(* Logix 5000 AddOnInstructionDefinition export CIP_Axis_Disable; software revision 34.01 *)

TYPE CIP_Axis :   // CIP Sync Axis Object
STRUCT
   Control : CIP_Control;   // Control bits to send to the drive
   Status : CIP_Status;   // Status bits received from the drive
   Input : CIP_AxisInputData;   // Data from the drive
   Output : CIP_AxisOutputData;   // Data to the drive
   PositionFeedback : DINT;   // Actual Position Value
   PositionCommand : DINT;   // Drive's commanded position
   ResponseTimestamp : LINT;   // Drive's timestamp of response
   RequestedAction : INT;   // State_Machine_Requested_Action
END_STRUCT
END_TYPE

TYPE CIP_AxisInputData :
STRUCT
   Data : SINT[10];
END_STRUCT
END_TYPE

TYPE CIP_AxisOutputData :
STRUCT
   Data : SINT[14];
END_STRUCT
END_TYPE

TYPE CIP_Control :
STRUCT
   Switch_On : BOOL;
   Disable_Voltage : BOOL;
   Quick_Stop : BOOL;
   Enable_Operation : BOOL;
   Op_Mode_Specific_4 : BOOL;   // Home Start or Follow Position bit, depending on on whether bit 11 (Mode Home) or bit 12 (C
   Op_Mode_Specific_5 : BOOL;   // Unused
   Op_Mode_Specific_6 : BOOL;   // Unused
   Reset_Fault : BOOL;
   Pause_Halt : BOOL;
   Op_Mode_Specific_9 : BOOL;   // Unused
   Reserved_10 : BOOL;
   Manu_Specific_11 : BOOL;   // Mode Home bit
   Manu_Specific_12 : BOOL;   // Mode Cyclic Position bit
   Manu_Specific_13 : BOOL;   // Unused
   Manu_Specific_14 : BOOL;   // Unused
   Manu_Specific_15 : BOOL;   // Unused
END_STRUCT
END_TYPE

TYPE CIP_DynamicMap :
STRUCT
   Input : CIP_MapInputData;   // Map data from the drive
   Output : CIP_MapOutputData;   // Map data to the drive
END_STRUCT
END_TYPE

TYPE CIP_MapInputData :   // Map data received from the drive
STRUCT
   Data : SINT[40];
END_STRUCT
END_TYPE

TYPE CIP_MapOutputData :   // Map data going to drive
STRUCT
   Data : SINT[32];
END_STRUCT
END_TYPE

TYPE CIP_Status :   // All connections to the drive ethernet module are established and data is successfully transferring.
STRUCT
   Ready_To_Switch_On : BOOL;
   Switched_On : BOOL;
   Operation_Enabled : BOOL;
   Fault : BOOL;
   Voltage_Enabled : BOOL;
   Quick_Stop : BOOL;
   Switch_On_Disabled : BOOL;
   Warning : BOOL;
   STO_Active : BOOL;
   Remote : BOOL;
   Target_Reached : BOOL;
   Internal_Limit_Active : BOOL;
   Op_Mode_Specific_12 : BOOL;   // Home Attained bit
   Op_Mode_Specific_13 : BOOL;   // Homing/Cyclic Position Error bit
   Manu_Specific_14 : BOOL;   // Motion Mode bit (0 for Homing, 1 for Cyclic Position)
   Manu_Specific_15 : BOOL;   // Following Position bit (for Cyclic Position mode)
END_STRUCT
END_TYPE

ADD_ON_INSTRUCTION CIP_Axis_Disable   (* revision 2.1, ExecutePrescan, ExecuteEnableInFalse *)
// Disable CIP Sync Axis
VAR_OUTPUT
   DN : BOOL; {access Read Only, visible}   // Command Successful
   ER : BOOL; {access Read Only, visible}   // Error
END_VAR
VAR_IN_OUT
   Axis : CIP_Axis; {required}
END_VAR
VAR_OUTPUT
   Error_Code : SINT; {access Read Only, visible}
END_VAR
VAR_IN_OUT
   Error_Description : STRING; {required}
END_VAR
VAR
   CommandTimeout : TIMER;   // Timeout Timer
   Step : SINT; {access None}
   ErrorEnumeratedValues : STRING[2] := ([0] := 'No Error', [1] := 'Command Timeout'); {access None}
END_VAR

ROUTINE EnableInFalse   (* ladder *)
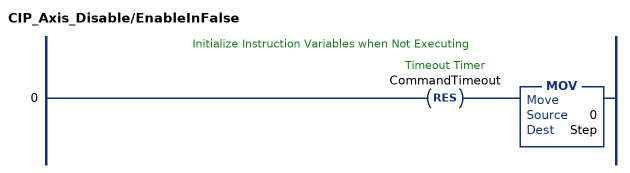
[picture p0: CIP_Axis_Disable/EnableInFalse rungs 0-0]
   // Initialize Instruction Variables when Not Executing
   0: RES(CommandTimeout)MOV(0,Step);
END_ROUTINE

ROUTINE Logic   (* ladder *)
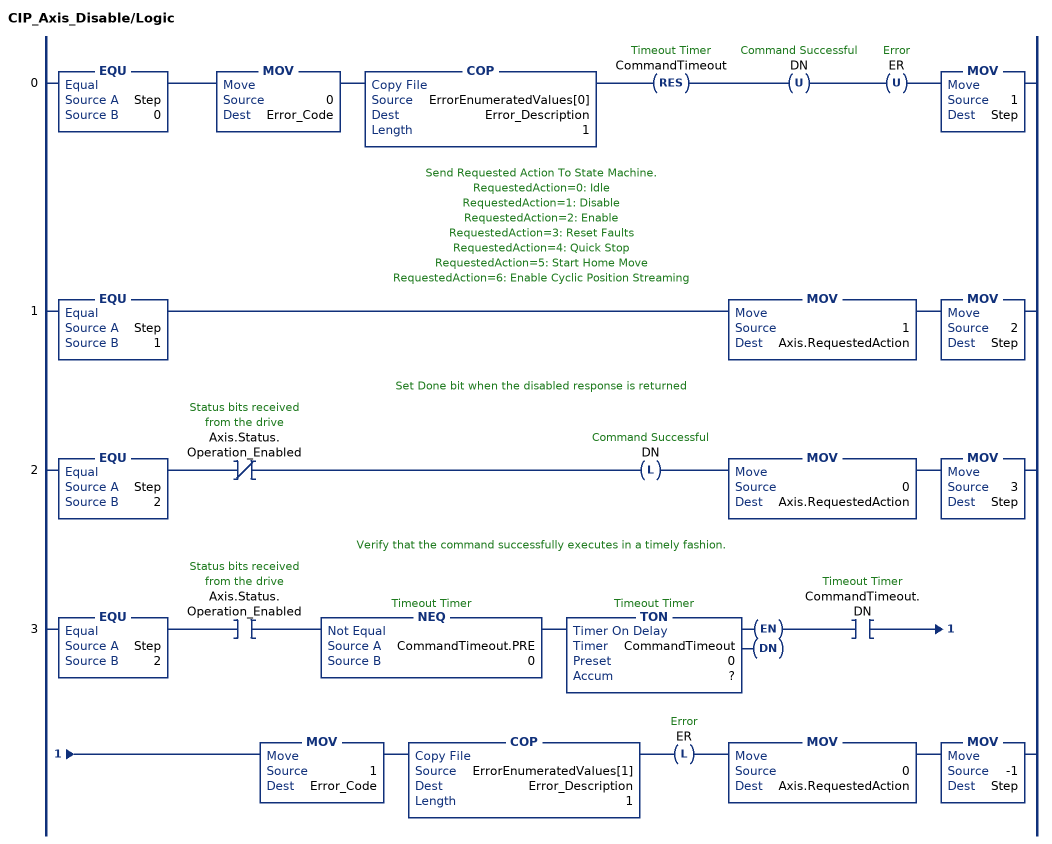
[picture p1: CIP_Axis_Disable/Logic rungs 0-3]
   0: EQU(Step,0)MOV(0,Error_Code)COP(ErrorEnumeratedValues[0],Error_Description,1)RES(CommandTimeout)OTU(DN)OTU(ER)MOV(1,Step);
   // Send Requested Action To State Machine.
   // RequestedAction=0: Idle
   // RequestedAction=1: Disable
   // RequestedAction=2: Enable
   // RequestedAction=3: Reset Faults
   // RequestedAction=4: Quick Stop
   // RequestedAction=5: Start Home Move
   // RequestedAction=6: Enable Cyclic Position Streaming
   1: EQU(Step,1)MOV(1,Axis.RequestedAction)MOV(2,Step);
   // Set Done bit when the disabled response is returned
   2: EQU(Step,2)XIO(Axis.Status.Operation_Enabled)OTL(DN)MOV(0,Axis.RequestedAction)MOV(3,Step);
   // Verify that the command successfully executes in a timely fashion.
   3: EQU(Step,2)XIC(Axis.Status.Operation_Enabled)NEQ(CommandTimeout.PRE,0)TON(CommandTimeout,?,?)XIC(CommandTimeout.DN)MOV(1,Error_Code)COP(ErrorEnumeratedValues[1],Error_Description,1)OTL(ER)MOV(0,Axis.RequestedAction)MOV(-1,Step);
END_ROUTINE

ROUTINE Prescan   (* ladder *)
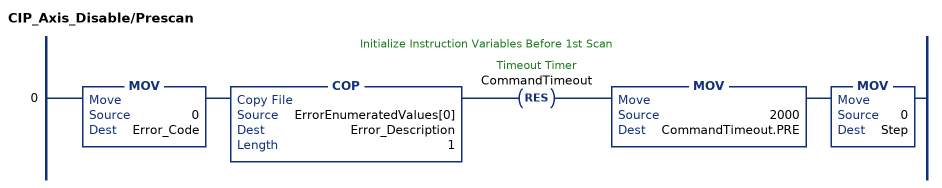
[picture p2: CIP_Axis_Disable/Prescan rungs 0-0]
   // Initialize Instruction Variables Before 1st Scan
   0: MOV(0,Error_Code)COP(ErrorEnumeratedValues[0],Error_Description,1)RES(CommandTimeout)MOV(2000,CommandTimeout.PRE)MOV(0,Step);
END_ROUTINE
END_ADD_ON_INSTRUCTION

ADD_ON_INSTRUCTION CIP_Axis_Disable_Streaming   (* revision 2.1, ExecutePrescan, ExecuteEnableInFalse *)
// CIP Sync Axis Disable Streaming
VAR_OUTPUT
   DN : BOOL; {access Read Only, visible}   // Command Successful
   ER : BOOL; {access Read Only, visible}   // Error
END_VAR
VAR_IN_OUT
   Axis : CIP_Axis; {required}
END_VAR
VAR_OUTPUT
   Error_Code : SINT; {access Read Only, visible}
END_VAR
VAR_IN_OUT
   Error_Description : STRING; {required}
END_VAR
VAR
   CommandTimeout : TIMER := (PRE := 2000); {access None}   // Timeout Timer
   Step : SINT; {access None}
   ErrorEnumeratedValues : STRING[2] := ([0] := 'No Error', [1] := 'Command Timeout'); {access None}
END_VAR

ROUTINE EnableInFalse   (* ladder *)
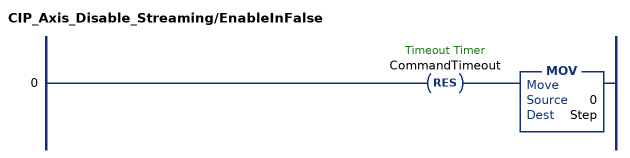
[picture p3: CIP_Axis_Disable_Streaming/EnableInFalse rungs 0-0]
   0: RES(CommandTimeout)MOV(0,Step);
END_ROUTINE

ROUTINE Logic   (* ladder *)
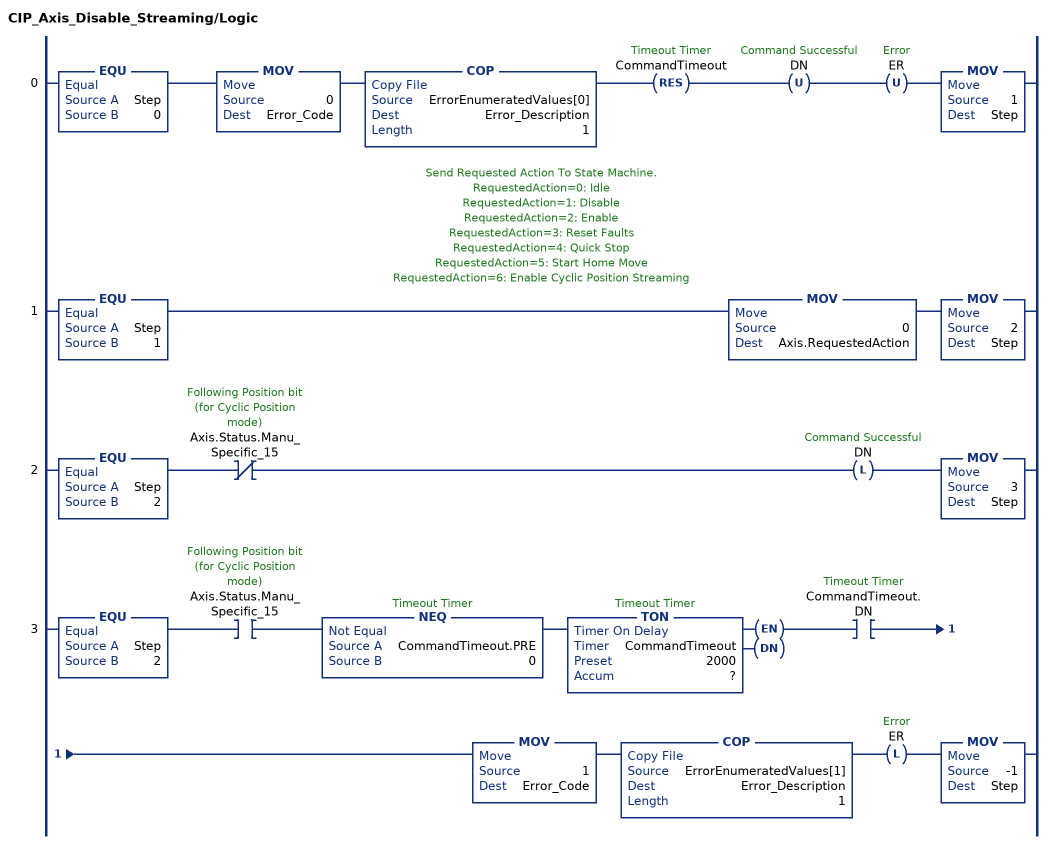
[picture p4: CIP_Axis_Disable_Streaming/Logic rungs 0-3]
   0: EQU(Step,0)MOV(0,Error_Code)COP(ErrorEnumeratedValues[0],Error_Description,1)RES(CommandTimeout)OTU(DN)OTU(ER)MOV(1,Step);
   // Send Requested Action To State Machine.
   // RequestedAction=0: Idle
   // RequestedAction=1: Disable
   // RequestedAction=2: Enable
   // RequestedAction=3: Reset Faults
   // RequestedAction=4: Quick Stop
   // RequestedAction=5: Start Home Move
   // RequestedAction=6: Enable Cyclic Position Streaming
   1: EQU(Step,1)MOV(0,Axis.RequestedAction)MOV(2,Step);
   2: EQU(Step,2)XIO(Axis.Status.Manu_Specific_15)OTL(DN)MOV(3,Step);
   3: EQU(Step,2)XIC(Axis.Status.Manu_Specific_15)NEQ(CommandTimeout.PRE,0)TON(CommandTimeout,?,?)XIC(CommandTimeout.DN)MOV(1,Error_Code)COP(ErrorEnumeratedValues[1],Error_Description,1)OTL(ER)MOV(-1,Step);
END_ROUTINE

ROUTINE Prescan   (* ladder *)
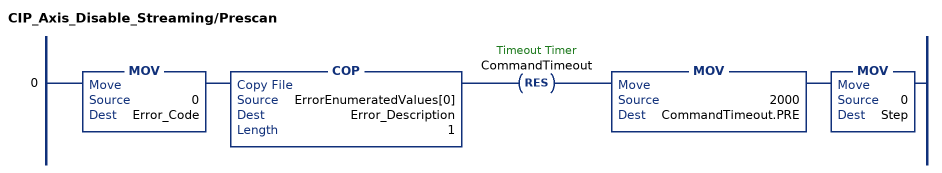
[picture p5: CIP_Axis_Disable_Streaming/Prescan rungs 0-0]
   0: MOV(0,Error_Code)COP(ErrorEnumeratedValues[0],Error_Description,1)RES(CommandTimeout)MOV(2000,CommandTimeout.PRE)MOV(0,Step);
END_ROUTINE
END_ADD_ON_INSTRUCTION

ADD_ON_INSTRUCTION CIP_Axis_Enable   (* revision 2.1, ExecutePrescan, ExecuteEnableInFalse *)
// Enables CIP Sync Axis
// Revision note:
// Bugfix: Added check of Axis.Status.Quick_Stop bit for confirming completion
VAR_OUTPUT
   DN : BOOL; {access Read Only, visible}   // Command Successful
   ER : BOOL; {access Read Only, visible}   // Error
END_VAR
VAR_IN_OUT
   Axis : CIP_Axis; {required}
END_VAR
VAR_OUTPUT
   Error_Code : SINT; {access Read Only, visible}
END_VAR
VAR_IN_OUT
   Error_Description : STRING; {required}
END_VAR
VAR
   CommandTimeout : TIMER := (PRE := 2000);   // Timeout Timer
   Step : SINT; {access None}
   ErrorEnumeratedValues : STRING[3] := ([0] := 'No Error', [1] := 'Command Timeout', [2] := 'Axis Faulted'); {access None}
END_VAR

ROUTINE EnableInFalse   (* ladder *)
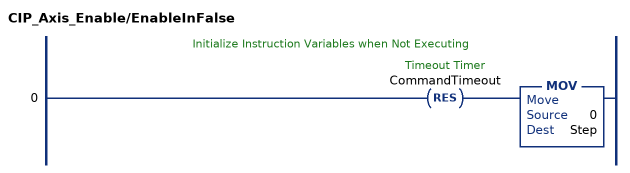
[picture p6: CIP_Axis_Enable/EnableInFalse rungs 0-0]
   // Initialize Instruction Variables when Not Executing
   0: RES(CommandTimeout)MOV(0,Step);
END_ROUTINE

ROUTINE Logic   (* ladder *)
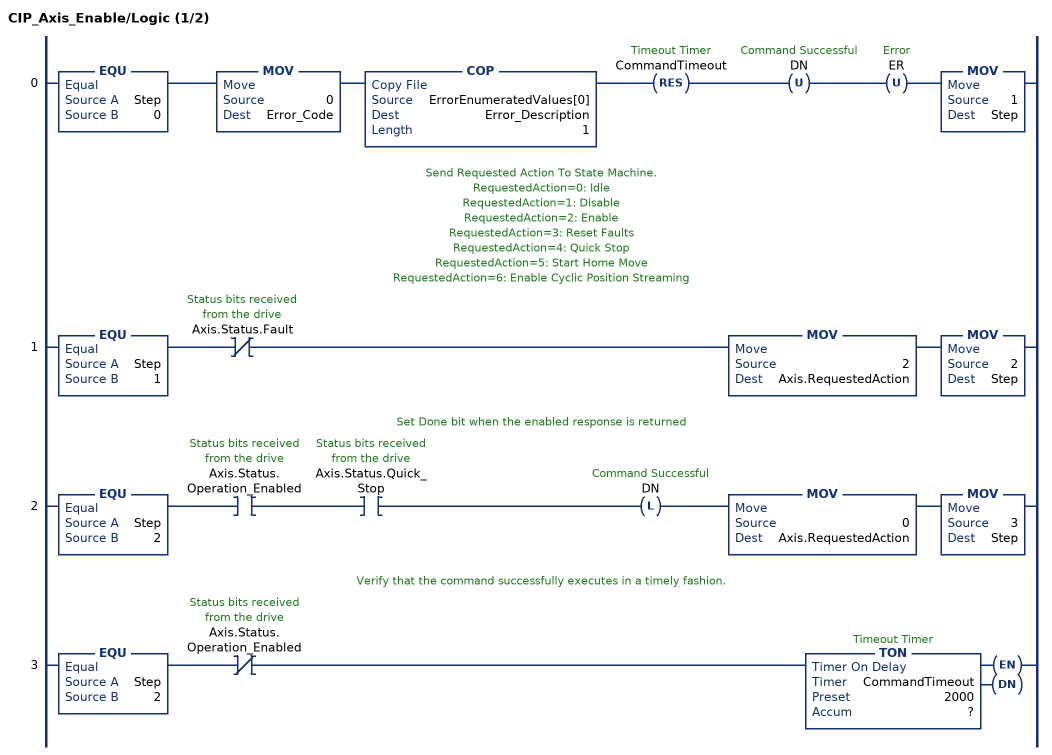
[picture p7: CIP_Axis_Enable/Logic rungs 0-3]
   0: EQU(Step,0)MOV(0,Error_Code)COP(ErrorEnumeratedValues[0],Error_Description,1)RES(CommandTimeout)OTU(DN)OTU(ER)MOV(1,Step);
   // Send Requested Action To State Machine.
   // RequestedAction=0: Idle
   // RequestedAction=1: Disable
   // RequestedAction=2: Enable
   // RequestedAction=3: Reset Faults
   // RequestedAction=4: Quick Stop
   // RequestedAction=5: Start Home Move
   // RequestedAction=6: Enable Cyclic Position Streaming
   1: EQU(Step,1)XIO(Axis.Status.Fault)MOV(2,Axis.RequestedAction)MOV(2,Step);
   // Set Done bit when the enabled response is returned
   2: EQU(Step,2)XIC(Axis.Status.Operation_Enabled)XIC(Axis.Status.Quick_Stop)OTL(DN)MOV(0,Axis.RequestedAction)MOV(3,Step);
   // Verify that the command successfully executes in a timely fashion.
   3: EQU(Step,2)XIO(Axis.Status.Operation_Enabled)TON(CommandTimeout,?,?);
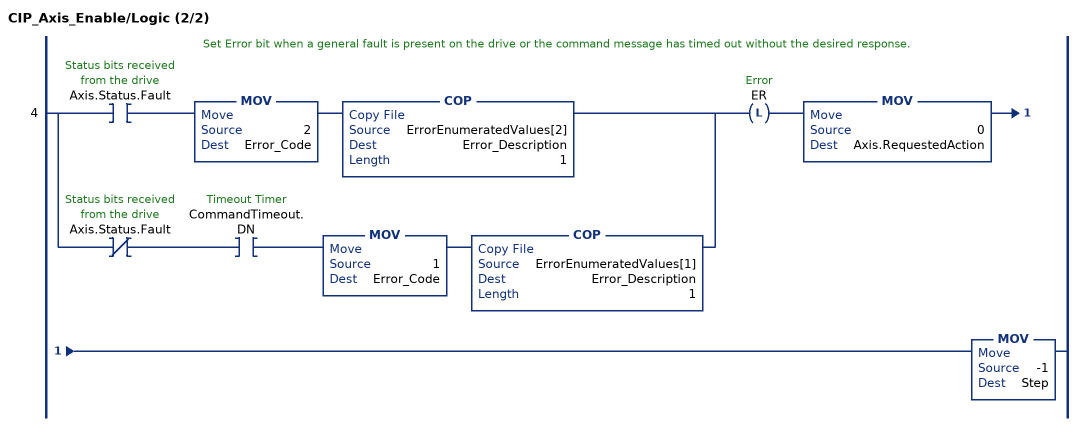
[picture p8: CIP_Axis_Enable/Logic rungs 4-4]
   // Set Error bit when a general fault is present on the drive or the command message has timed out without the desired response.
   4: [XIC(Axis.Status.Fault) MOV(2,Error_Code) COP(ErrorEnumeratedValues[2],Error_Description,1) ,XIO(Axis.Status.Fault) XIC(CommandTimeout.DN) MOV(1,Error_Code) COP(ErrorEnumeratedValues[1],Error_Description,1) ]OTL(ER)MOV(0,Axis.RequestedAction)MOV(-1,Step);
END_ROUTINE

ROUTINE Prescan   (* ladder *)
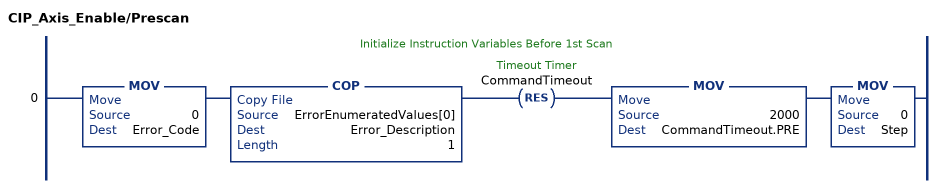
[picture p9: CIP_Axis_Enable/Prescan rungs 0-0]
   // Initialize Instruction Variables Before 1st Scan
   0: MOV(0,Error_Code)COP(ErrorEnumeratedValues[0],Error_Description,1)RES(CommandTimeout)MOV(2000,CommandTimeout.PRE)MOV(0,Step);
END_ROUTINE
END_ADD_ON_INSTRUCTION

ADD_ON_INSTRUCTION CIP_Axis_Enable_Streaming   (* revision 2.1, ExecutePrescan, ExecuteEnableInFalse *)
// CIP Sync Axis Enable Streaming
VAR_OUTPUT
   DN : BOOL; {access Read Only, visible}   // Command Successful
   ER : BOOL; {access Read Only, visible}   // Error
END_VAR
VAR_IN_OUT
   Axis : CIP_Axis; {required}
END_VAR
VAR_OUTPUT
   Error_Code : SINT; {visible}
END_VAR
VAR_IN_OUT
   Error_Description : STRING; {required}
END_VAR
VAR
   CommandTimeout : TIMER := (PRE := 2000); {access None}   // Timeout Timer
   Step : SINT; {access None}
   ErrorEnumeratedValues : STRING[5] := ([0] := 'No Error', [1] := 'Command Timeout', [2] := 'Axis Faulted', [3] := 'Home Not Attained', [4] := 'Axis Not Enabled'); {access None}
END_VAR

ROUTINE EnableInFalse   (* ladder *)
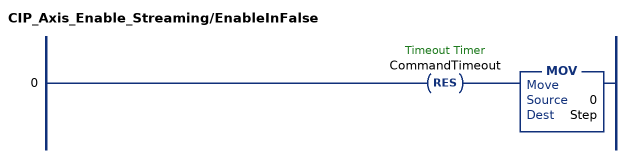
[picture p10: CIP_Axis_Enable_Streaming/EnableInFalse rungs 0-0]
   0: RES(CommandTimeout)MOV(0,Step);
END_ROUTINE

ROUTINE Logic   (* ladder *)
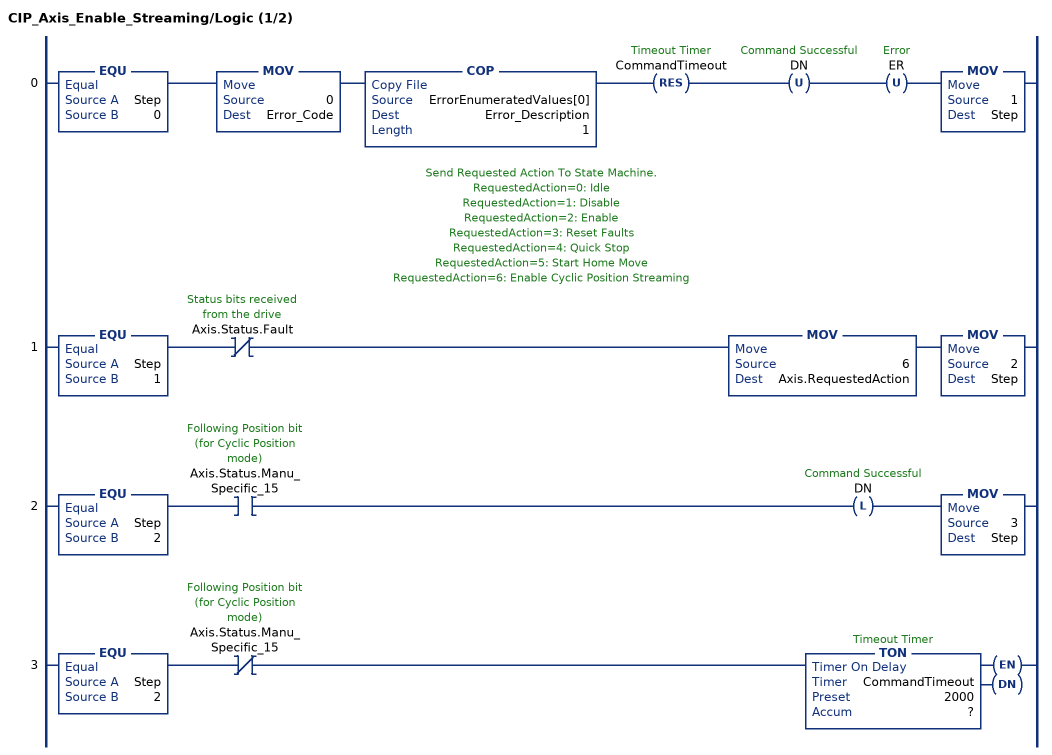
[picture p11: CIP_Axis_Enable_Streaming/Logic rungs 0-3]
   0: EQU(Step,0)MOV(0,Error_Code)COP(ErrorEnumeratedValues[0],Error_Description,1)RES(CommandTimeout)OTU(DN)OTU(ER)MOV(1,Step);
   // Send Requested Action To State Machine.
   // RequestedAction=0: Idle
   // RequestedAction=1: Disable
   // RequestedAction=2: Enable
   // RequestedAction=3: Reset Faults
   // RequestedAction=4: Quick Stop
   // RequestedAction=5: Start Home Move
   // RequestedAction=6: Enable Cyclic Position Streaming
   1: EQU(Step,1)XIO(Axis.Status.Fault)MOV(6,Axis.RequestedAction)MOV(2,Step);
   2: EQU(Step,2)XIC(Axis.Status.Manu_Specific_15)OTL(DN)MOV(3,Step);
   3: EQU(Step,2)XIO(Axis.Status.Manu_Specific_15)TON(CommandTimeout,?,?);
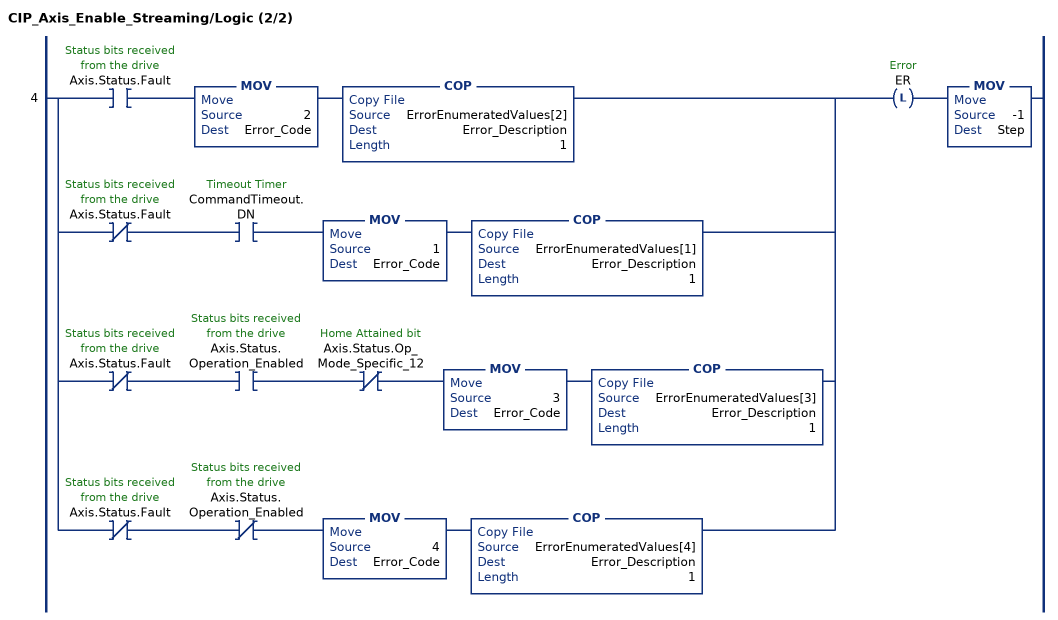
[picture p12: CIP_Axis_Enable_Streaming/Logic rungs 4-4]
   4: [XIC(Axis.Status.Fault) MOV(2,Error_Code) COP(ErrorEnumeratedValues[2],Error_Description,1) ,XIO(Axis.Status.Fault) XIC(CommandTimeout.DN) MOV(1,Error_Code) COP(ErrorEnumeratedValues[1],Error_Description,1) ,XIO(Axis.Status.Fault) XIC(Axis.Status.Operation_Enabled) XIO(Axis.Status.Op_Mode_Specific_12) MOV(3,Error_Code) COP(ErrorEnumeratedValues[3],Error_Description,1) ,XIO(Axis.Status.Fault) XIO(Axis.Status.Operation_Enabled) MOV(4,Error_Code) COP(ErrorEnumeratedValues[4],Error_Description,1) ]OTL(ER)MOV(-1,Step);
END_ROUTINE

ROUTINE Prescan   (* ladder *)
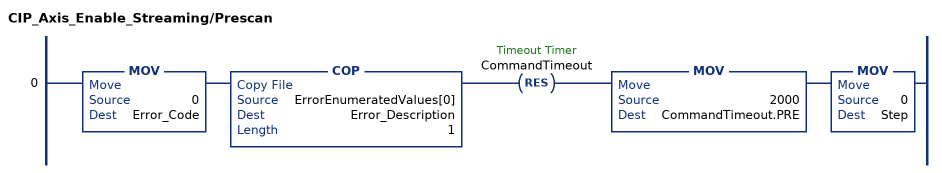
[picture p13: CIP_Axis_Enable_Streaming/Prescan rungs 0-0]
   0: MOV(0,Error_Code)COP(ErrorEnumeratedValues[0],Error_Description,1)RES(CommandTimeout)MOV(2000,CommandTimeout.PRE)MOV(0,Step);
END_ROUTINE
END_ADD_ON_INSTRUCTION

ADD_ON_INSTRUCTION CIP_Axis_Fault_Reset   (* revision 2.1, ExecutePrescan, ExecuteEnableInFalse *)
// CIP Sync Axis Fault Reset
VAR_OUTPUT
   DN : BOOL; {access Read Only, visible}   // Command Successful
   ER : BOOL; {access Read Only, visible}   // Error
END_VAR
VAR_IN_OUT
   Axis : CIP_Axis; {required}
END_VAR
VAR_OUTPUT
   Error_Code : SINT; {access Read Only, visible}
END_VAR
VAR_IN_OUT
   Error_Description : STRING; {required}
END_VAR
VAR
   Step : SINT;
   CommandTimeout : TIMER := (PRE := 2000); {access None}
   ErrorEnumeratedValues : STRING[2] := ([0] := 'No Error', [1] := 'Command Timeout'); {access None}
END_VAR

ROUTINE EnableInFalse   (* ladder *)
// EnableIn_False
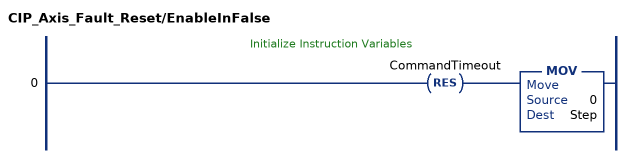
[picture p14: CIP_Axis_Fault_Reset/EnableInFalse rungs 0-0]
   // Initialize Instruction Variables
   0: RES(CommandTimeout)MOV(0,Step);
END_ROUTINE

ROUTINE Logic   (* ladder *)
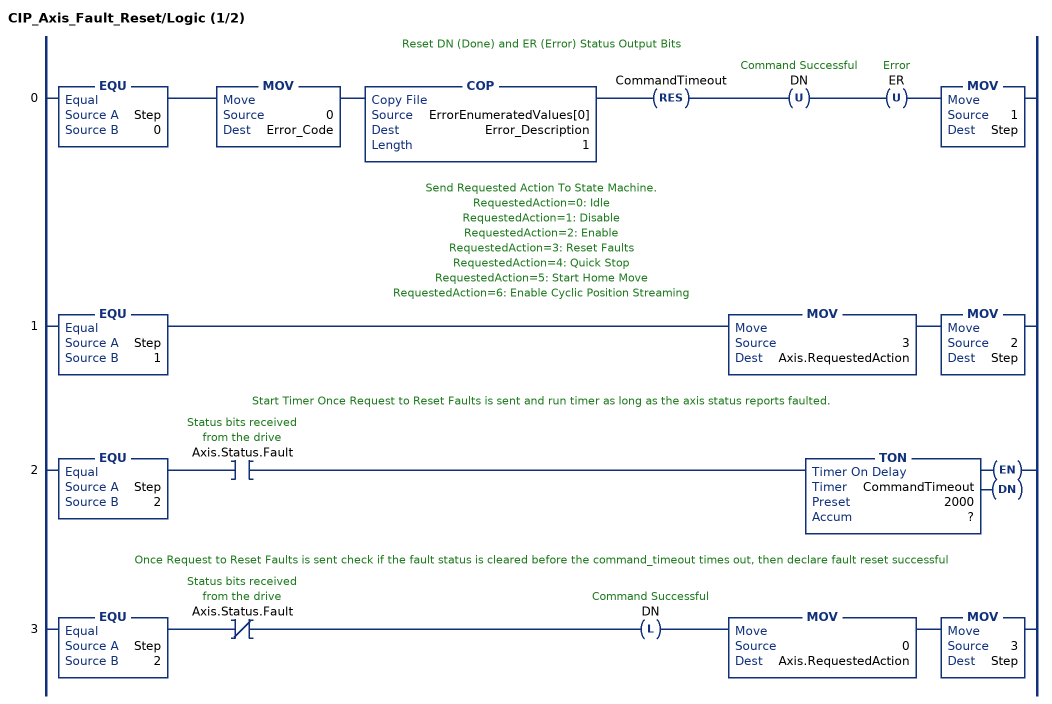
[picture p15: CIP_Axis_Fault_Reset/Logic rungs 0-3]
   // Reset DN (Done) and ER (Error) Status Output Bits
   0: EQU(Step,0)MOV(0,Error_Code)COP(ErrorEnumeratedValues[0],Error_Description,1)RES(CommandTimeout)OTU(DN)OTU(ER)MOV(1,Step);
   // Send Requested Action To State Machine.
   // RequestedAction=0: Idle
   // RequestedAction=1: Disable
   // RequestedAction=2: Enable
   // RequestedAction=3: Reset Faults
   // RequestedAction=4: Quick Stop
   // RequestedAction=5: Start Home Move
   // RequestedAction=6: Enable Cyclic Position Streaming
   1: EQU(Step,1)MOV(3,Axis.RequestedAction)MOV(2,Step);
   // Start Timer Once Request to Reset Faults is sent and run timer as long as the axis status reports faulted.
   2: EQU(Step,2)XIC(Axis.Status.Fault)TON(CommandTimeout,?,?);
   // Once Request to Reset Faults is sent check if the fault status is cleared before the command_timeout times out, then declare fault reset successful
   3: EQU(Step,2)XIO(Axis.Status.Fault)OTL(DN)MOV(0,Axis.RequestedAction)MOV(3,Step);
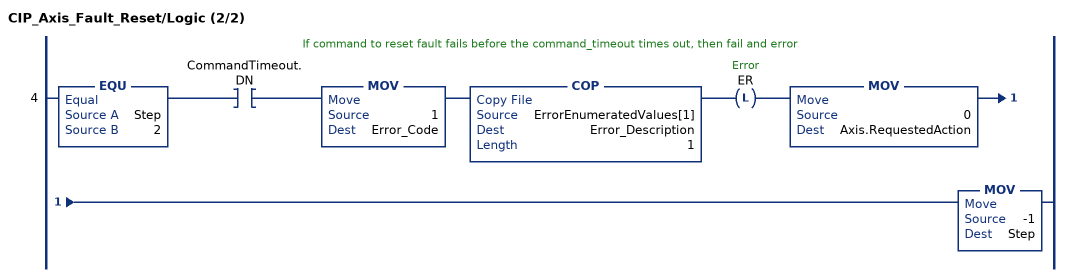
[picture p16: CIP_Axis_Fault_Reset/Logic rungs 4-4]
   // If command to reset fault fails before the command_timeout times out, then fail and error
   4: EQU(Step,2)XIC(CommandTimeout.DN)MOV(1,Error_Code)COP(ErrorEnumeratedValues[1],Error_Description,1)OTL(ER)MOV(0,Axis.RequestedAction)MOV(-1,Step);
END_ROUTINE

ROUTINE Prescan   (* ladder *)
// Prescan
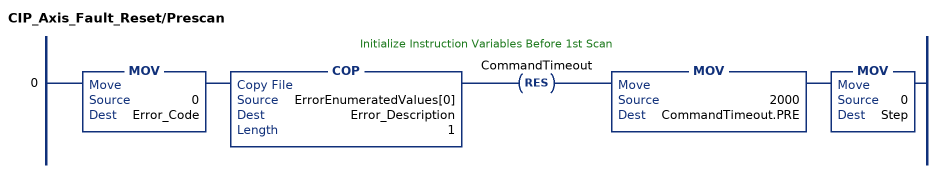
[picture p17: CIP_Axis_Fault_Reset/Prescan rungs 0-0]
   // Initialize Instruction Variables Before 1st Scan
   0: MOV(0,Error_Code)COP(ErrorEnumeratedValues[0],Error_Description,1)RES(CommandTimeout)MOV(2000,CommandTimeout.PRE)MOV(0,Step);
END_ROUTINE
END_ADD_ON_INSTRUCTION
